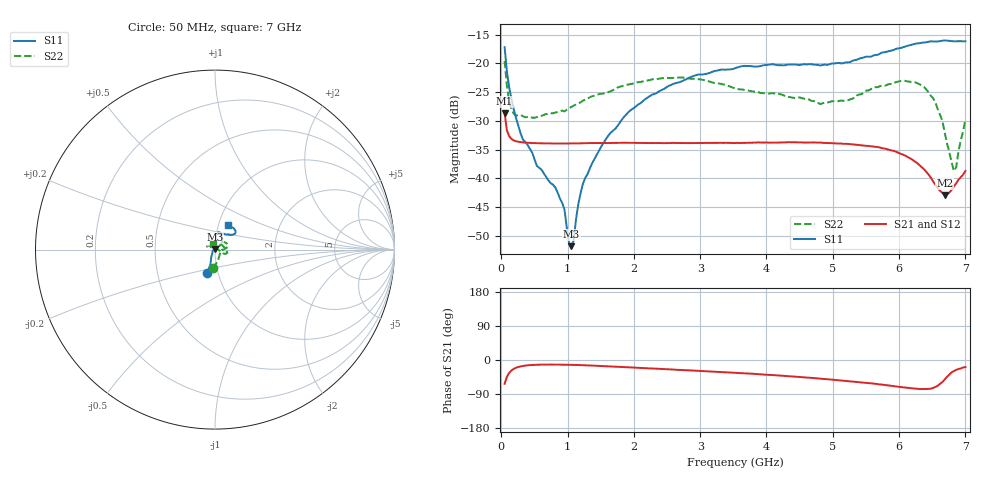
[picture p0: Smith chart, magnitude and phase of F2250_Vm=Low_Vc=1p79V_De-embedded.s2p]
! Integrated Device Technology
! Corporate Headquarters
! 6024 Silver Creek Valley Road
! San Jose, CA 95138  USA
! Phone:  1-408-284-8200
! Toll Free:  1-800-223-1366
! Webpage:  http://www.idt.com/
! Timing and RF Division
! 515 Groton Road, Suite 102
! Westford, MA 01886-6024
! Device:  F2250
! Description: Voltage Variable RF Attenuator
! Frequency:  50.0 -  6000.00 MHz
! Package:  3x3 mm Thin QFN Plastic Package: 16 pin
! Ports:  2 RF, 3 DC
!  Pin  1  = GND
!  Pin  2  = NC
!  Pin  3  = RF1  = Port 1
!  Pin  4  = NC
!  Pin  5  = GND
!  Pin  6  = GND
!  Pin  7  = GND
!  Pin  8  = GND
!  Pin  9  = NC
!  Pin 10  = RF2  = Port 2
!  Pin 11  = NC
!  Pin 12  = GND
!  Pin 13  = GND
!  Pin 14  = VCNTRL
!  Pin 15  = VDD
!  Pin 16  = VMODE
! Vcntrl:  1.790 Volts
! Vmode:  +0.000 Volts
! Vdd:  +3.30  Volts
! Current:  1.185 mA
! Data:  The device was measured on a the F2250 evaluation board which has
!  individual transmission lines to the RF pins.  Data was collected
!  using a calibrated network analyzer.  The evaluation board was
!  de-embedded using a TRL calibration technique.
!  The reference plane is the edge of the package pin.
! Misc:  SN 10
!  Action Tracker AT0258
! Date Measured:  2014-11-26
! Date:  2015-10-15  MJV
! Note:
!  Integrated Device Technology supplies this data as a sample of measured
!  data at the package pin for this product.  Your particular data for this
!  product may vary.
!  Data was taken at 25 degrees C.
!  Integrated Device Technology reserves the right to change this data at anytime.
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# GHz S dB R 50
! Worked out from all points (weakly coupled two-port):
!   201 points, 50 MHz to 7 GHz, reference 50 ohm
!   highest |S21| = -28.65 dB at 50 MHz (marker M1); lowest = -43.0 dB at 6.687 GHz (marker M2)
!   lowest |S11| = -51.8 dB at 1.058 GHz (marker M3), VSWR 1.01, Z = 49.9 + j0.229 ohm
!   |S11| at or under -10 dB: start of sweep to end of sweep
!   |S22| runs from -38.7 to -19.6 dB; largest |S21 - S12| = 5.5e-05
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0.05  -17.17 -108.3  -28.65 -62.8  -28.65 -62.8  -19.56 -96.3
0.1195  -24.20 -111.3  -32.68 -33.9  -32.68 -33.9  -26.60 -61.6
0.22375  -29.55 -121.4  -33.54 -20.4  -33.54 -20.4  -29.04 -37.2
0.5365  -37.81 -154.3  -33.87 -12.5  -33.87 -12.5  -29.33 -8.5
0.91875  -44.26 157.9  -33.94 -12.3  -33.93 -12.4  -28.20 -4.2
0.9535  -45.44 169.9  -33.93 -12.4  -33.92 -12.4  -28.35 -2.9
1.023  -51.36 141.5  -33.92 -12.6  -33.93 -12.7  -27.78 -0.9
1.05775  -51.79 116.7  -33.92 -12.8  -33.92 -12.8  -27.57 -0.3
1.0925  -50.77 81.1  -33.91 -12.9  -33.90 -12.9  -27.34 -0.7
1.2315  -40.91 41.5  -33.88 -13.7  -33.87 -13.6  -26.49 -1.3
1.6485  -32.06 40.9  -33.84 -16.8  -33.84 -16.8  -24.84 5.9
2.37825  -24.87 46.9  -33.84 -23.3  -33.86 -23.3  -22.66 16.4
3.525  -20.83 72.2  -33.85 -33.8  -33.84 -33.9  -24.35 42.5
4.7065  -20.20 72.2  -33.74 -47.6  -33.75 -47.6  -26.54 49.8
5.22775  -19.81 56.2  -34.00 -55.6  -33.99 -55.6  -26.39 23.2
5.85325  -17.84 40.3  -35.04 -67.5  -35.03 -67.5  -23.58 -7.1
6.3745  -16.35 41.3  -38.39 -76.7  -38.40 -76.7  -24.10 -21.4
6.54825  -16.20 45.0  -41.09 -71.0  -41.11 -71.0  -26.82 -24.0
6.68725  -16.00 48.7  -42.96 -51.3  -42.97 -51.1  -31.97 -10.8
6.82625  -16.15 53.4  -41.39 -29.1  -41.35 -29.0  -38.70 48.0
6.861  -16.14 55.0  -40.87 -26.0  -40.83 -26.1  -38.09 68.0
7  -16.14 63.2  -38.70 -18.7  -38.67 -18.8  -29.81 113.5
